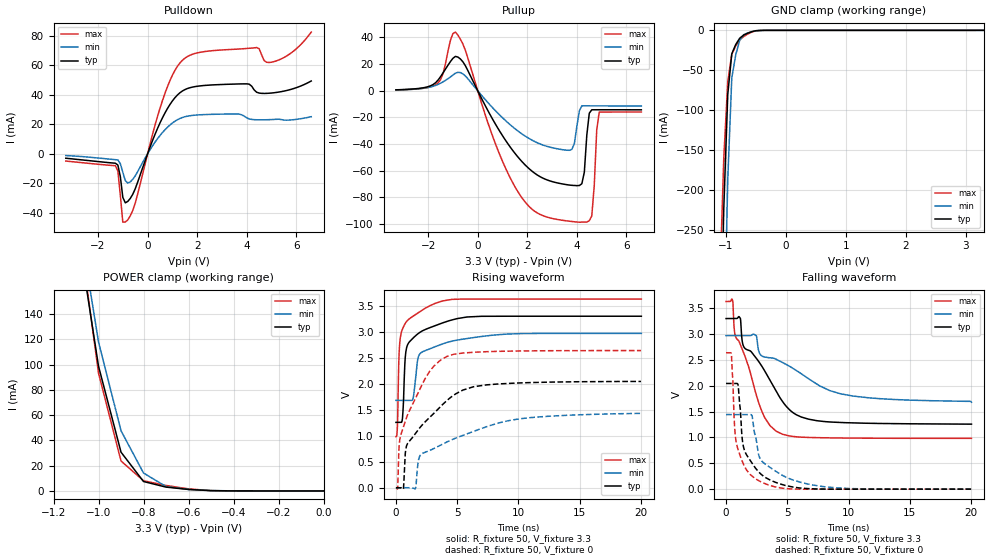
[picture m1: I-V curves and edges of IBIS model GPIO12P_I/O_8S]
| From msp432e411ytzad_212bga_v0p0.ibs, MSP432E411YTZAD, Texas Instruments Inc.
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|   Model Cell GPIO12P_I/O_8S
[Model]   GPIO12P_I/O_8S
Model_type   I/O
Polarity   Non-Inverting
Enable   Active-Low
Vinl =  0.8
Vinh =  2
Cref =  15.0000pF
Rref =  100.0000M
Vref =  0V
Vmeas =  1.65
C_comp   6.029616p   5.226915p   6.778838p
[Model Spec]
Vinl   0.8   0.8   0.8
Vinh   2   2   2
[Temperature Range]   25   125   -40
[Voltage Range]   3.3   2.97   3.63
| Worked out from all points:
|   slope of the pulldown table from 0 to 0.495 V, typ, clamps not added: 23.8 ohm
|   slope of the pullup table from 0 to 0.495 V, typ, clamps not added: 27.8 ohm
|   GND clamp passes 1 mA (typ) near -0.53 V on its own axis
|   POWER clamp passes 1 mA (typ) near -0.58 V on its own axis
|   rising waveform, R_fixture 50, V_fixture 3.3: 20-80 % time 834ps typ, 1.66ns min, 464ps max; typ from 1.26 V to 3.3 V
|   rising waveform, R_fixture 50, V_fixture 0: 20-80 % time 3.27ns typ, 5.48ns min, 2.21ns max; typ from 0 V to 2.04 V
|   falling waveform, R_fixture 50, V_fixture 3.3: 20-80 % time 3.4ns typ, 5.55ns min, 2.25ns max; typ from 3.3 V to 1.26 V
|   falling waveform, R_fixture 50, V_fixture 0: 20-80 % time 1.28ns typ, 2.16ns min, 784ps max; typ from 2.04 V to 0 V
| Nom Voltages:
|   IBIASFET=3.3, VDDC=1.2, VDD=3.3, GND=0
| Min Voltages:
|   IBIASFET=2.97, VDDC=1.08, VDD=2.97, GND=0
| Max Voltages:
|   IBIASFET=3.63, VDDC=1.32, VDD=3.63, GND=0
[POWER_clamp]
|   voltage   I(typ)   I(min)   I(max)
-3.3V     3.668A     4.187A     4.057A
-1.067V   175.6mA    191.7mA    181.3mA
-1.033V   137.2mA    154.7mA    137.2mA
-1V       98.66mA    117.8mA    93.17mA
-900mV    30.66mA    47.6mA     23.68mA
-800mV    7.454mA    14.17mA    8.045mA
-700mV    3.021mA    3.466mA    4.326mA
-600mV    1.166mA    1.15mA     1.613mA
-500mV    219.7uA    295.1uA    245.5uA
0V        69.07pA    1.982nA    9.028pA
[Pulldown]
|   voltage   I(typ)   I(min)   I(max)
-3.3V     -3.019mA   -1.206mA   -4.938mA
-1.3V     -6.416mA   -4.007mA   -8.087mA
-1.2V     -7.65mA    -4.163mA   -11.69mA
-1V       -29.59mA   -12.56mA   -46.46mA
-900mV    -33.29mA   -18.21mA   -46.32mA
-500mV    -23.81mA   -14.98mA   -33.54mA
700mV     27.72mA    16.29mA    41.06mA
1.4V      42.61mA    24.62mA    63.44mA
4V        47.51mA    24.37mA    71.53mA
4.4V      41.79mA    23.1mA     72.14mA
5V        41.27mA    23.24mA    62.2mA
6.6V      49.45mA    25.19mA    82.65mA
[Pullup]
|   voltage   I(typ)   I(min)   I(max)
-3.3V     716.3uA    635uA      605.7uA
-1.6V     8.021mA    4.755mA    5.925mA
-900mV    25.8mA     13.18mA    44.03mA
1.7V      -51.4mA    -31.27mA   -78.06mA
3.7V      -70.75mA   -44.67mA   -97.88mA
4V        -71.18mA   -26.4mA    -98.48mA
4.3V      -61.06mA   -11.3mA    -98.51mA
4.5V      -16.84mA   -11.31mA   -97.48mA
4.6V      -14.26mA   -11.32mA   -93.92mA
4.8V      -14.25mA   -11.33mA   -29.37mA
4.9V      -14.25mA   -11.34mA   -16.02mA
6.6V      -14.3mA    -11.49mA   -15.93mA
[GND_clamp]
|   voltage   I(typ)   I(min)   I(max)
-3.3V     -18.01A    -17.27A    -18.6A
-1.1V     -459.9mA   -734.3mA   -318.7mA
-1.033V   -223.6mA   -411.6mA   -160.4mA
-966.7mV  -80.12mA   -186.8mA   -64.21mA
-900mV    -29.51mA   -59.8mA    -30.11mA
-833.3mV  -17.66mA   -30.4mA    -19.41mA
-766.7mV  -9.785mA   -12.28mA   -11.96mA
-700mV    -5.884mA   -5.445mA   -7.749mA
-500mV    -484.3uA   -573uA     -552.3uA
-366.7mV  -23.48uA   -48.41uA   -21.82uA
3.3V      69.07pA    6.412uA    7.794pA
[Ramp]
| variable   typ   min   max
dV/dt_f  1.2484834/3.3898513n 0.79075867/5.5201485n  1.6167624/2.2426289n
dV/dt_r  1.2448904/3.2567253n 0.88403346/5.4513958n  1.5995284/2.1976543n
R_load = 50
[Rising Waveform]
R_fixture = 50
V_fixture = 3.3
V_fixture_min = 2.97
V_fixture_max = 3.63
|   time   V(typ)   V(min)   V(max)
0s        1.258V     1.681V     982.5mV
112.1ps   1.258V     1.681V     1.123V
249ps     1.258V     1.681V     2.527V
410.6ps   1.256V     1.681V     2.957V
550.4ps   1.382V     1.681V     3.061V
880.4ps   2.702V     1.681V     3.202V
1.389ns   2.877V     1.707V     3.299V
1.811ns   2.965V     2.5V       3.366V
2.361ns   3.041V     2.635V     3.449V
20.04ns   3.3V       2.97V      3.63V
[Rising Waveform]
R_fixture = 50
V_fixture = 0
V_fixture_min = 0
V_fixture_max = 0
|   time   V(typ)   V(min)   V(max)
0s        0V         0V         0V
137.5ps   0V         0V         -10.27mV
285.5ps   0V         0V         867.9mV
608.8ps   -19.72mV   0V         1.164V
751.6ps   625.5mV    0V         1.271V
946.3ps   849.3mV    0V         1.399V
1.591ns   1.043V     -19.71mV   1.715V
2.053ns   1.183V     642.2mV    1.945V
4.184ns   1.682V     883.5mV    2.529V
20.01ns   2.045V     1.447V     2.639V
[Falling Waveform]
R_fixture = 50
V_fixture = 3.3
V_fixture_min = 2.97
V_fixture_max = 3.63
|   time   V(typ)   V(min)   V(max)
0s        3.3V       2.97V      3.63V
536.6ps   3.3V       2.97V      3.649V
710.7ps   3.3V       2.97V      3.017V
1.152ns   3.31V      2.97V      2.806V
1.45ns    2.753V     2.97V      2.631V
2.471ns   2.533V     2.968V     1.821V
2.918ns   2.381V     2.578V     1.508V
4.094ns   1.897V     2.512V     1.121V
7.391ns   1.325V     2.037V     996.4mV
20.04ns   1.258V     1.681V     982.8mV
[Falling Waveform]
R_fixture = 50
V_fixture = 0
V_fixture_min = 0
V_fixture_max = 0
|   time   V(typ)   V(min)   V(max)
0s        2.045V     1.443V     2.639V
436.5ps   2.045V     1.443V     2.606V
695.2ps   2.045V     1.443V     1.218V
904.8ps   2.045V     1.443V     826.9mV
1.001ns   1.981V     1.443V     750.7mV
1.42ns    822.5mV    1.443V     483.8mV
2.11ns    507.6mV    1.425V     255.9mV
2.62ns    343.6mV    706.6mV    169.6mV
6.996ns   7.379mV    84.18mV    0V
20.01ns   0V         0V         0V
